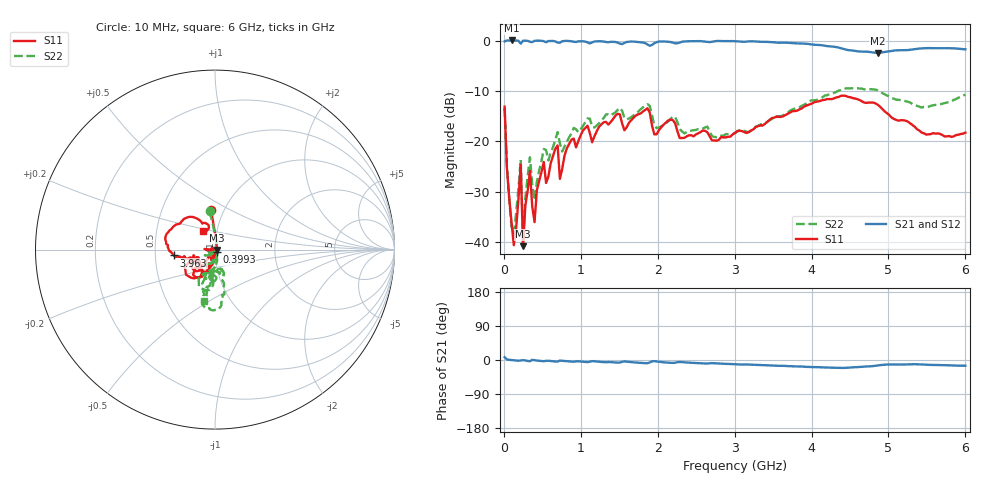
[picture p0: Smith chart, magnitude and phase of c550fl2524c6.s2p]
!Agilent Technologies,N5234A,MY52241123,A.10.00.00
!Agilent N5234A: A.10.00.00
!Date: Wednesday, March 20, 2019 09:48:31
!Correction: S11(Full 2 Port(1,2))
!S21(Full 2 Port(1,2))
!S12(Full 2 Port(1,2))
!S22(Full 2 Port(1,2))
!S2P File: Measurements: S11, S21, S12, S22:
# Hz S  dB  R 50
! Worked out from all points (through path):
!   201 points, 10 MHz to 6 GHz, reference 50 ohm
!   highest |S21| = 0.07 dB at 99.85 MHz (marker M1); lowest = -2.4 dB at 4.862 GHz (marker M2)
!   group delay of S21, straight-line fit = 7.86 ps
!   lowest |S11| = -40.8 dB at 249.6 MHz (marker M3), VSWR 1.02, Z = 50.9 - j0.264 ohm
!   |S11| at or under -10 dB: start of sweep to end of sweep
!   |S22| runs from -40.1 to -9.4 dB; largest |S21 - S12| = 0.0052
!   S11 on the Smith chart (normalised r, x): 10 MHz: 0.87, +0.40; 399.4 MHz: 1.02, -0.03; 3.963 GHz: 0.63, -0.04; 6 GHz: 0.85, +0.18
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1e7  -13.10 95.6  -0.12 7.4  -0.14 7.4  -13.36 97.9
3.995e7  -25.29 83.6  0.07 1.5  0.07 1.4  -25.02 82.4
9.985e7  -36.11 52.3  0.07 -0.1  0.07 -0.1  -36.95 43.7
1.298e8  -40.65 3.2  0.07 -0.6  0.06 -0.5  -38.28 -11.6
2.1965e8  -24.64 176.6  -0.57 -1.0  -0.58 -1.0  -23.64 -150.8
2.496e8  -40.84 -16.6  0.01 -0.4  0.01 -0.4  -40.13 -70.7
3.3945e8  -25.84 -121.1  -0.19 -3.4  -0.20 -3.3  -23.16 -96.5
3.9935e8  -36.05 -56.0  -0.00 -0.7  0.00 -0.8  -31.70 -91.9
4.293e8  -29.71 -73.8  0.03 -1.5  0.06 -1.5  -28.02 -80.1
5.1915e8  -24.09 -108.9  -0.07 -3.2  -0.09 -3.2  -21.52 -85.7
5.491e8  -28.27 -131.7  -0.28 -2.1  -0.27 -2.1  -21.73 -109.0
6.9885e8  -20.81 -126.7  -0.37 -4.3  -0.36 -4.3  -18.15 -102.8
7.288e8  -27.45 -135.5  -0.37 -1.5  -0.38 -1.5  -20.39 -122.5
1.0283e9  -17.84 -109.1  -0.10 -4.7  -0.13 -4.6  -16.98 -95.7
1.8669e9  -13.41 -139.0  -0.72 -8.4  -0.71 -8.3  -12.61 -103.6
2.01665e9  -17.77 -128.4  -0.16 -4.6  -0.16 -4.9  -17.21 -98.5
3.005e9  -18.35 -155.2  -0.08 -11.3  -0.08 -11.4  -18.29 -69.4
3.9634e9  -12.71 -171.9  -0.63 -18.3  -0.63 -18.3  -12.14 -77.7
4.0233e9  -12.32 -175.9  -0.76 -18.8  -0.77 -18.6  -11.83 -79.6
4.8619e9  -12.72 127.8  -2.39 -14.3  -2.39 -14.5  -9.86 -101.4
5.01165e9  -14.78 117.0  -2.08 -11.8  -2.07 -11.8  -11.10 -104.4
6e9  -18.25 124.2  -1.70 -15.1  -1.70 -15.2  -10.70 -101.8
